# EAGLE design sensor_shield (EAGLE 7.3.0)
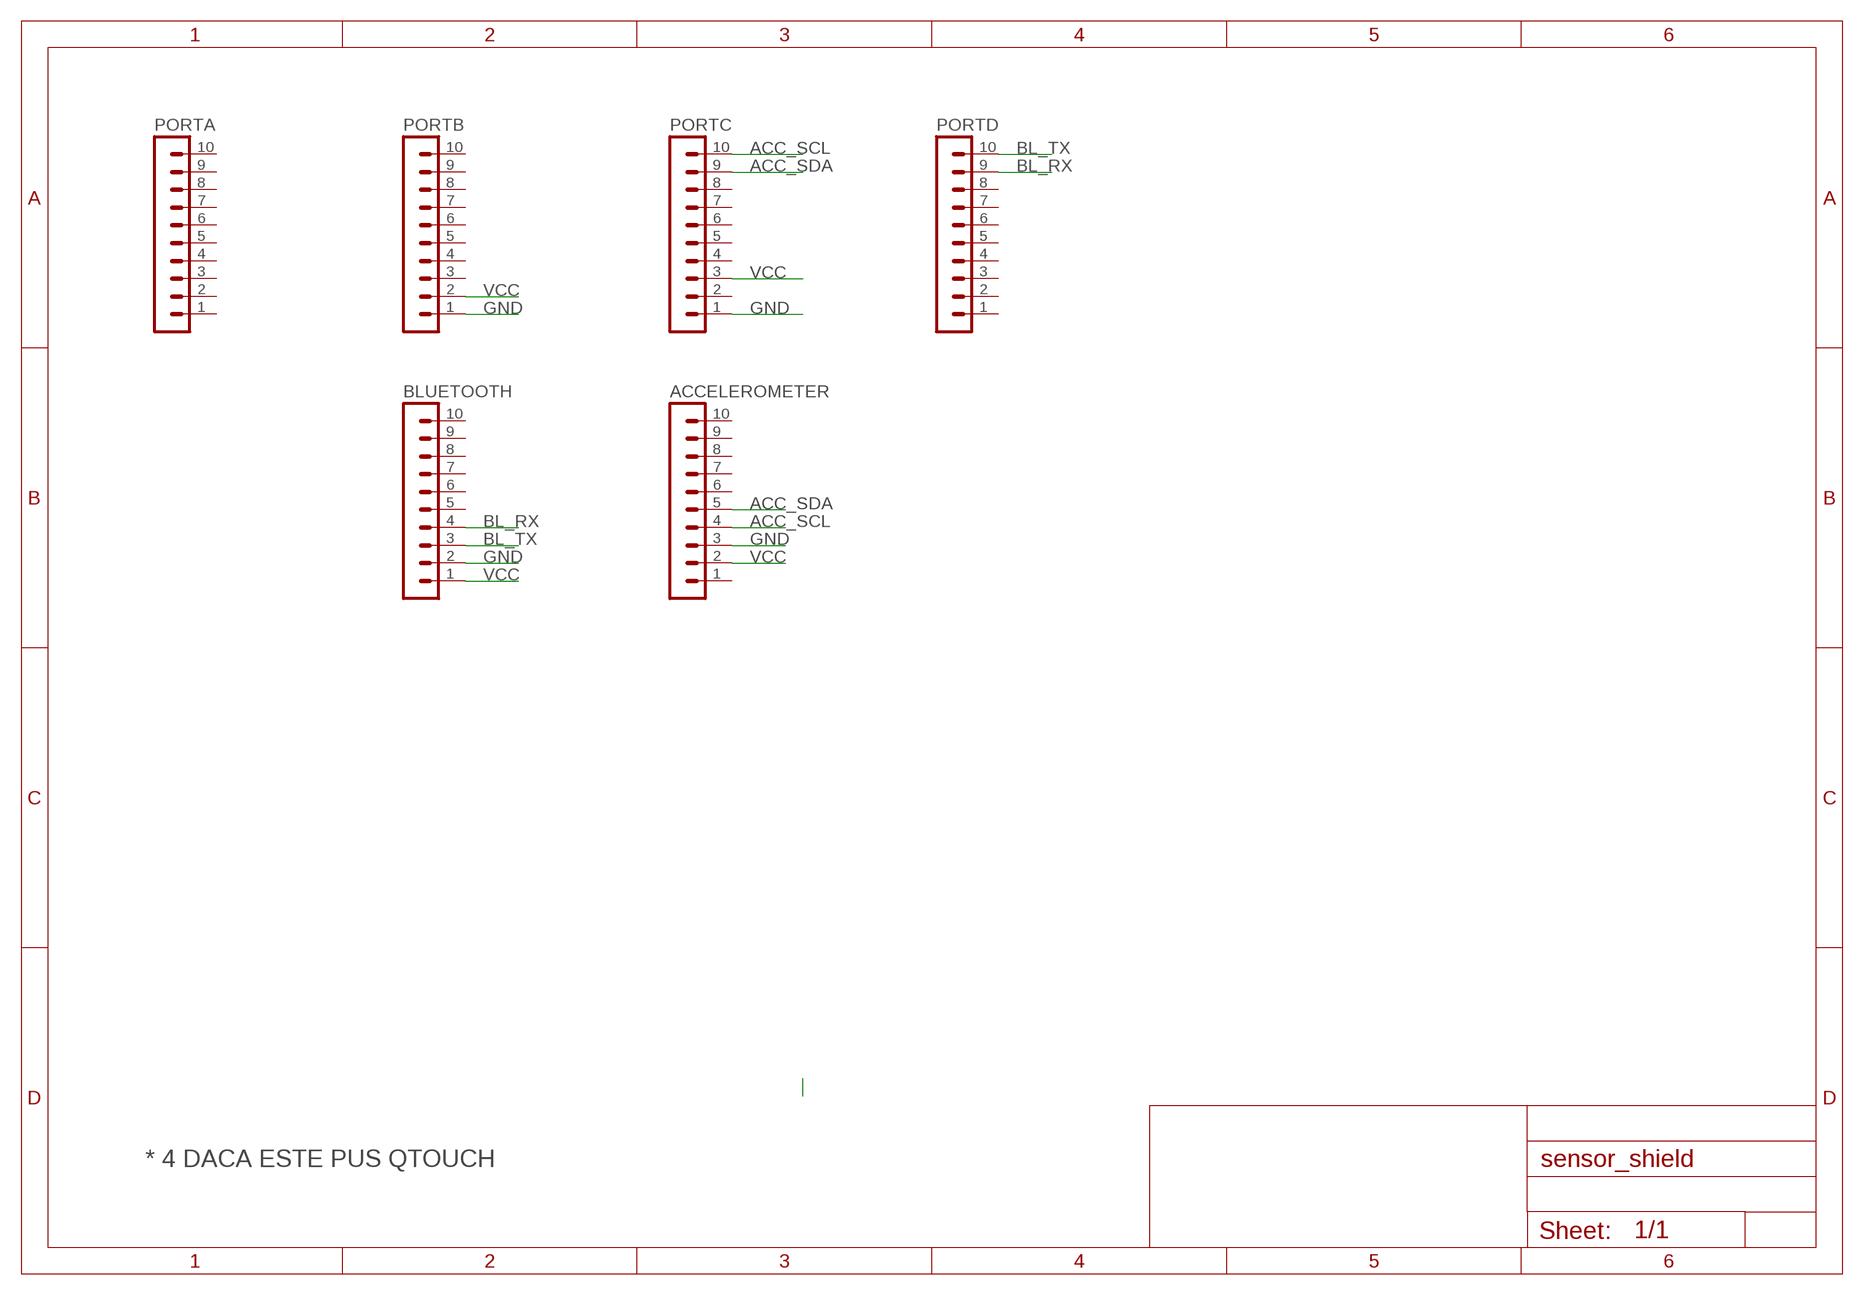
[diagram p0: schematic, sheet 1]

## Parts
ACCELEROMETER  MA10-1  [MA10-1]
BLUETOOTH  MA10-1  [MA10-1]
PORTA  MA10-1  [MA10-1]
PORTB  MA10-1  [MA10-1]
PORTC  MA10-1  [MA10-1]
PORTD  MA10-1  [MA10-1]

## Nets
ACC_SCL: ACCELEROMETER.4 PORTC.10
ACC_SDA: ACCELEROMETER.5 PORTC.9
BL_RX: BLUETOOTH.4 PORTD.9
BL_TX: BLUETOOTH.3 PORTD.10
GND: ACCELEROMETER.3 BLUETOOTH.2 PORTB.1 PORTC.1
VCC: ACCELEROMETER.2 BLUETOOTH.1 PORTB.2 PORTC.3
Unconnected: ACCELEROMETER.1 ACCELEROMETER.6 ACCELEROMETER.7 ACCELEROMETER.8 ACCELEROMETER.9 ACCELEROMETER.10 BLUETOOTH.5 BLUETOOTH.6 BLUETOOTH.7 BLUETOOTH.8 BLUETOOTH.9 BLUETOOTH.10 PORTA.1 PORTA.2 PORTA.3 PORTA.4 PORTA.5 PORTA.6 PORTA.7 PORTA.8 PORTA.9 PORTA.10 PORTB.3 PORTB.4 PORTB.5 PORTB.6 PORTB.7 PORTB.8 PORTB.9 PORTB.10 PORTC.2 PORTC.4 PORTC.5 PORTC.6 PORTC.7 PORTC.8 PORTD.1 PORTD.2 PORTD.3 PORTD.4 PORTD.5 PORTD.6 PORTD.7 PORTD.8

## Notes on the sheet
- * 4 DACA ESTE PUS QTOUCH

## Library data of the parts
ACCELEROMETER BLUETOOTH PORTA PORTB PORTC PORTD = con-lstb:MA10-1: PIN HEADER; OC_FARNELL: unknown; OC_NEWARK: unknown

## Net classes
1 power: width 0.61 mm

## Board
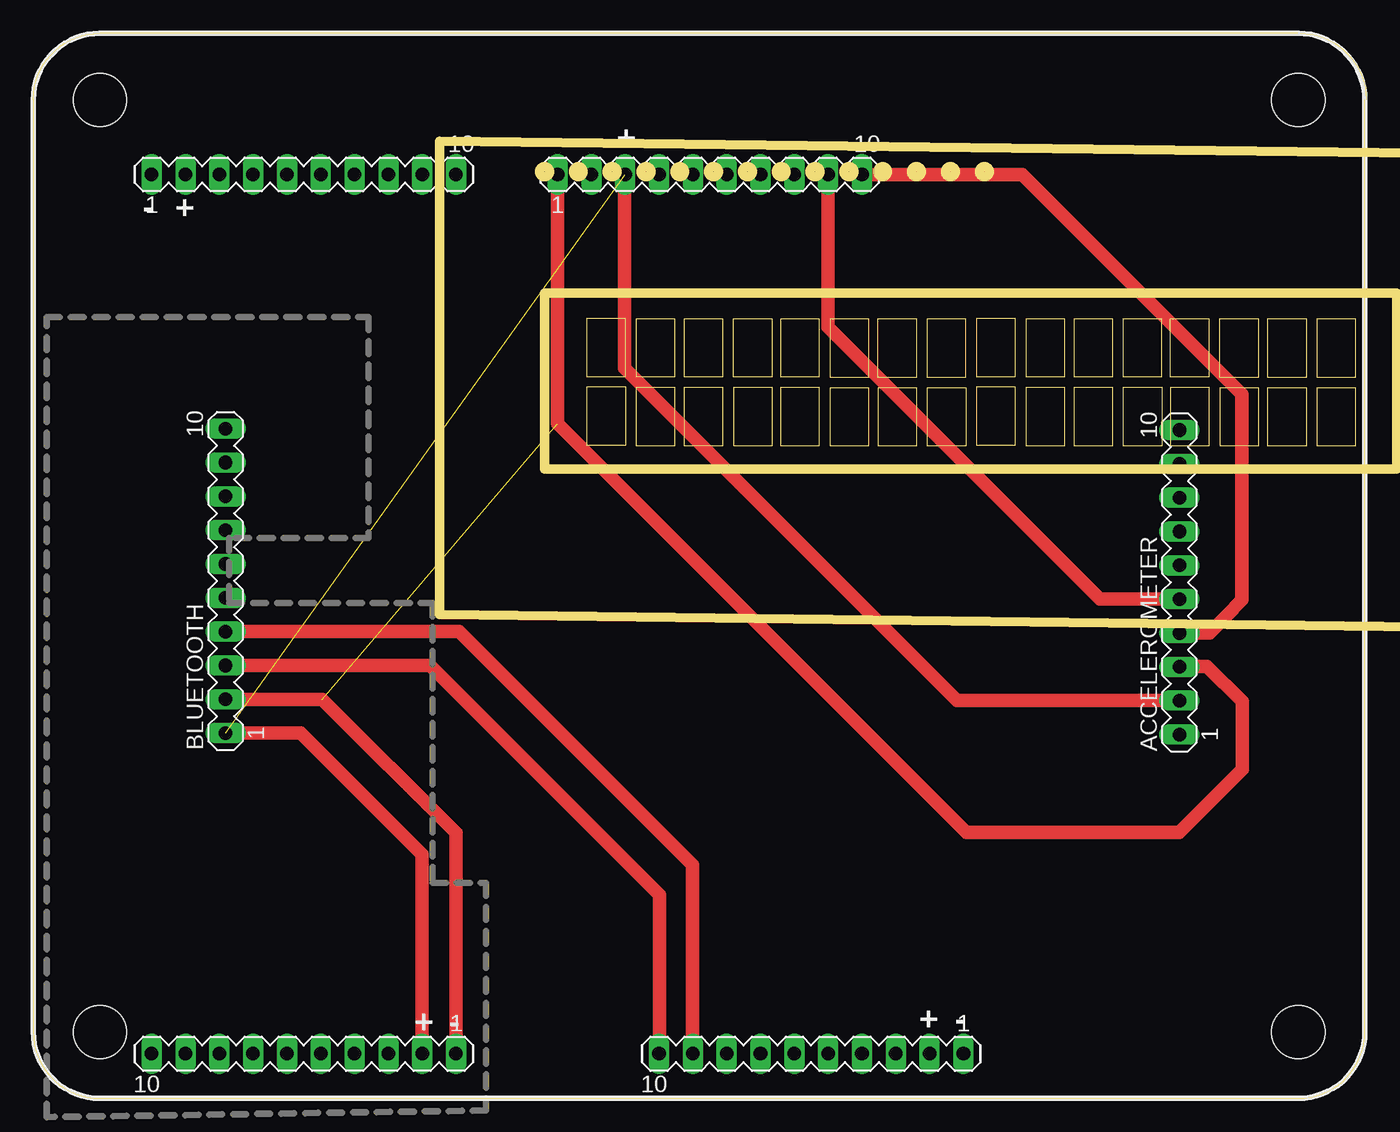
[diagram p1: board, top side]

Size 100.1 x 80 mm. Coordinates in mm from the lower left corner, seen from the top.
Outline: 100,75 100,5 arc-90 95,0 5,0 arc-90 0,5 0,75 arc-90 5,80 95,80
Outline: 95.1,80 arc-90 100.1,75
Copper layers (1*16): Top 0.035mm / dielectric 1.5mm / Bottom 0.035mm
Design rules "default": minimum track width 10mil, minimum drill 0.6mm, track to track 0.25mm, track to pad 10mil, pad to pad 0.2mm, via to via 10mil, smd to smd 0mil, copper to edge 40mil, drill to drill 10mil, minimum pad ring 10mil, minimum via ring 8mil, stop-mask expansion 0mil, vias tented up to drill 0mil, thermal gap 20mil
Holes 4 mm at 95,75 5,5 5,75 95,5
Milling: area 38,69.3 to 38.8,70; area 40.6,69.3 to 41.3,70; area 43.1,69.3 to 43.8,70; area 45.7,69.3 to 46.4,70; area 48.2,69.3 to 48.9,70; area 50.7,69.3 to 51.5,70; area 53.3,69.3 to 54,70; area 55.8,69.3 to 56.5,70; area 58.4,69.3 to 59.1,70; area 60.9,69.3 to 61.6,70; area 63.4,69.3 to 64.2,70; area 66,69.3 to 66.7,70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; 8 lines

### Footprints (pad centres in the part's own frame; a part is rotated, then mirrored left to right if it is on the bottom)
MA10-1 = drill 1.016 long: 1 -11.43,0; 2 -8.89,0; 3 -6.35,0; 4 -3.81,0; 5 -1.27,0; 6 1.27,0; 7 3.81,0; 8 6.35,0; 9 8.89,0; 10 11.43,0

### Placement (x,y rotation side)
ACCELEROMETER  86.07,38.77 90 top
BLUETOOTH  14.44,38.87 90 top
PORTA  20.32,69.4 0 top
PORTB  20.32,3.36 180 top
PORTC  50.8,69.4 0 top
PORTD  58.42,3.36 180 top

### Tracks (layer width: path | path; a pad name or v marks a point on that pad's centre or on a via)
ACC_SCL
  Top 0.406: 86.09,34.98 ACCELEROMETER.4
  Top 1.016: PORTC.10 74.29,69.4 90.77,52.89 90.76,37.42 88.36,34.97 ACCELEROMETER.4
ACC_SDA
  Top 0.406: 86.04,37.53 ACCELEROMETER.5
  Top 1.016: PORTC.9 59.69,57.94 80.11,37.52 86.05,37.52 ACCELEROMETER.5
BL_RX
  Top 0.406: 49.6,3.43 PORTD.9
  Top 1.016: BLUETOOTH.4 31.99,35.06 49.5,17.55 49.5,3.39 PORTD.9
BL_TX
  Top 0.406: 46.96,3.39 PORTD.10
  Top 1.016: BLUETOOTH.3 29.8,32.52 47.02,15.3 47.02,3.39 PORTD.10
GND  (1 unrouted)
  Top 0.406: 86.03,32.46 ACCELEROMETER.3 | 31.78,3.39 PORTB.1
  Top 1.016: PORTB.1 31.74,19.94 21.71,29.98 BLUETOOTH.2 | PORTC.1 39.37,50.67 70.06,19.98 86.05,19.98 90.78,24.71 90.78,29.81 88.14,32.46 86.11,32.46 ACCELEROMETER.3
VCC  (1 unrouted)
  Top 0.406: 86.14,29.81 ACCELEROMETER.2
  Top 1.016: BLUETOOTH.1 20.09,27.44 29.21,18.32 PORTB.2 | ACCELEROMETER.2 69.38,29.88 44.4,54.86 44.4,69.35 PORTC.3

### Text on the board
tNames: - | + | - | + | + | - | + | -
tDocu: Optional | alimentare 3.3V | Optional | alimentare 12V | Optional | QTouch
_bsilk: SJ1 | SJ2 | R10 | 100 | R11 | 100 | R14 | 100
215bmp: D:/Downloads/logo.bmp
